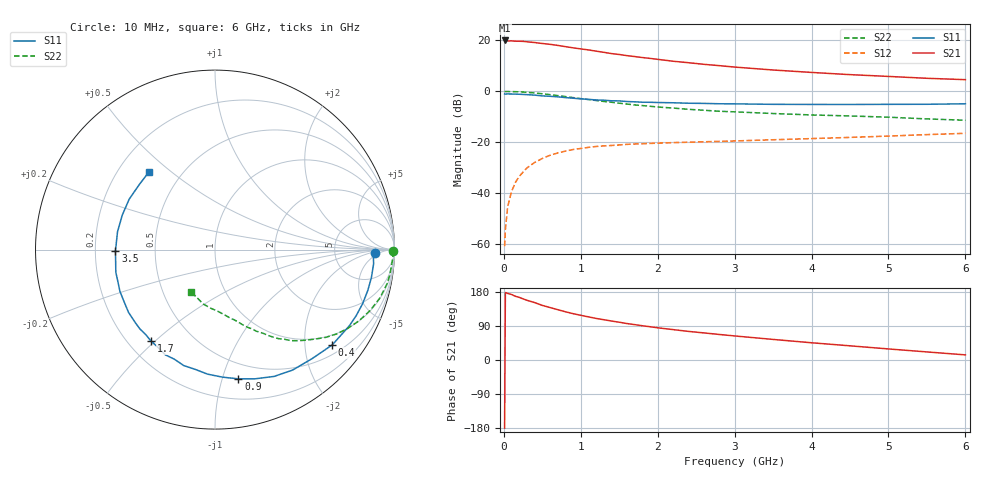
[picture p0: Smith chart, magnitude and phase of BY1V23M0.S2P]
! SIEMENS Small Signal Semiconductors
! BFY420
! Si NPN RF SIEGET Grounded Emitter Transistor in MICRO-X
! VCE = 1.25 V  IC = 3 mA
! Common Emitter S-Parameters:  October  1996
# GHz  S  MA  R  50
!  f  S11  S21  S12  S22
! GHz  MAG  ANG  MAG  ANG  MAG  ANG  MAG  ANG
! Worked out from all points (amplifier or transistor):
!   36 points, 10 MHz to 6 GHz, reference 50 ohm
!   highest |S21| = 20.0 dB at 10 MHz (marker M1)
!   |S21| within 3 dB of that: start of sweep to 923.6 MHz
!   unconditionally stable (mu >= 1): 3.595 GHz to end of sweep
!   at 250 MHz: K = 0.07, MSG = 25.7 dB, |S12| = -31.8 dB
!   at 1.4 GHz: K = 0.40, MSG = 18.1 dB, |S12| = -21.3 dB
!   at 6 GHz: K = 1.22, MAG = 7.7 dB, |S12| = -16.5 dB
!   S11 on the Smith chart (normalised r, x): 10 MHz: 17, -3; 400 MHz: 0.72, -2.64; 900 MHz: 0.36, -1.13; 1.7 GHz: 0.29, -0.48; 3.5 GHz: 0.29, -0.01; 6 GHz: 0.33, +0.42
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0.01  0.8894 -1.2  10.01 -179.7  0.0009 86.9  0.9939 -0.6
0.02  0.8827 -2.1  9.945 178.1  0.0019 85.9  0.9908 -1.0
0.05  0.8873 -5.1  9.781 175.7  0.0054 89.4  0.9919 -2.7
0.1  0.8852 -10.2  9.825 172.9  0.0107 86.5  0.9872 -5.6
0.15  0.8812 -14.9  9.68 168.2  0.0161 81.4  0.9833 -8.5
0.25  0.8685 -25.1  9.609 161.3  0.0258 76.0  0.9664 -13.8
0.3  0.8605 -29.6  9.426 157.6  0.0311 74.5  0.9565 -16.5
0.4  0.8418 -39.1  9.111 151.5  0.0399 67.7  0.9279 -21.5
0.5  0.8137 -48.2  8.726 144.1  0.0478 63.3  0.8952 -26.3
0.6  0.7984 -57.2  8.404 138.5  0.0552 59.1  0.86 -30.7
0.7  0.7796 -65.0  7.998 132.8  0.0613 55.1  0.8252 -34.7
0.9  0.7319 -79.7  7.168 122.3  0.0717 47.6  0.7523 -41.4
1.1  0.6951 -93.4  6.522 113.8  0.079 42.4  0.6887 -47.5
1.4  0.6511 -110.4  5.523 102.8  0.0861 35.9  0.6095 -54.5
1.7  0.6216 -125.1  4.828 93.4  0.0919 31.4  0.5403 -59.9
2  0.6024 -137.5  4.253 85.0  0.0956 28.1  0.4913 -64.5
2.2  0.5954 -144.0  3.908 80.2  0.0979 26.2  0.4688 -67.3
2.8  0.5694 -162.1  3.2 67.4  0.1036 22.9  0.4054 -74.7
3.5  0.5547 -179.3  2.627 54.3  0.1115 20.6  0.3659 -82.0
4.5  0.5512 159.5  2.129 37.4  0.1241 17.4  0.3277 -94.1
5.5  0.5562 139.3  1.804 21.3  0.1407 13.9  0.2866 -110.2
6  0.5685 130.1  1.696 13.5  0.1494 11.6  0.2699 -120.0
